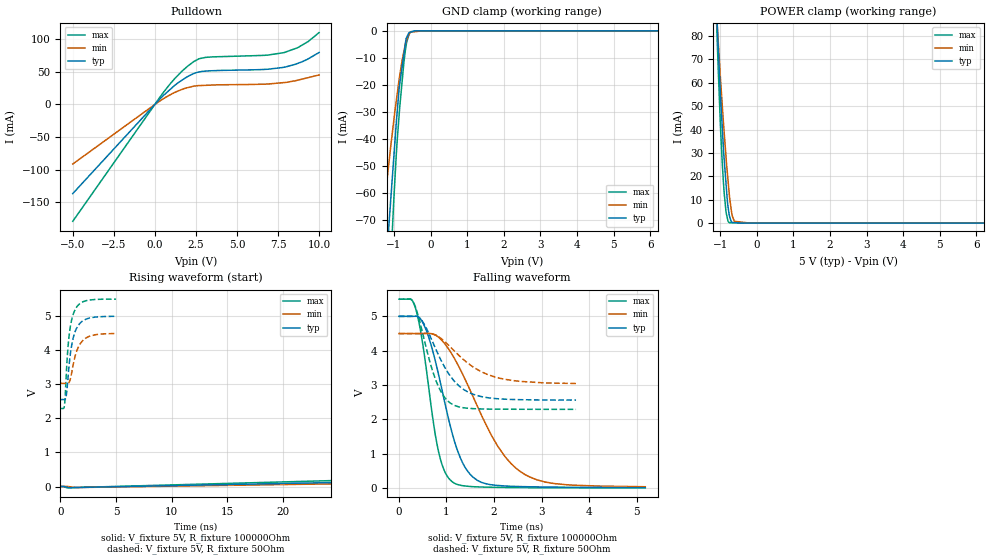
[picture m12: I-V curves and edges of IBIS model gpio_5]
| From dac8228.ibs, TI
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|   gpio_5 Model
[Model]   gpio_5
Model_type   I/O_open_drain
Polarity   Non-Inverting
Enable   Active-Low
Vinl = 0.8
Vinh = 3.8
Vmeas = 2.25
Vref = 5
Cref = 10pF
Rref = 100000
|   typ   min   max
|   (nom PVT)   (Fast PVT)   (slow PVT)
|C_comp from frequency method(F=50MHz)
|Average
C_comp   7.613e-12   6.267e-12   8.966e-12
|ON state : BUFFER OUTPUT TURNED LOW
|C_comp   7.719e-12   6.391e-12   9.083e-12
|OFF state: BUFFER IN HIGH IMPEDANCE
|C_comp   7.508e-12   6.143e-12   8.849e-12
|C_comp from L-C Tank method(L=1nH)
|Average
|C_comp   7.024e-12   5.919e-12   8.186e-12
|ON state : BUFFER OUTPUT TURNED LOW
|Resonant Frequency(Hz)   1.890e+09   2.050e+09   1.750e+09
|C_comp   7.098e-12   6.033e-12   8.279e-12
|OFF state: BUFFER IN HIGH IMPEDANCE
|Resonant Frequency(Hz)   1.910e+09   2.090e+09   1.770e+09
|C_comp   6.950e-12   5.805e-12   8.093e-12
| Where nom  PVT is Nominal Process,  5V,  33C
|   Fast PVT is Strong Process,   5.5V,  -40C
|   Slow PVT is Weak Process,   4.5V,  113C
[Voltage Range]   5   4.5   5.5
|Ambient Temperature   25   105   -40
|Junction Temperature
[Temperature Range]   33   113   -40
[Pullup Reference]   5   4.5   5.5
[Pulldown Reference]   0   0   0
[Power Clamp Reference]   5   4.5   5.5
[GND Clamp Reference]   0   0   0
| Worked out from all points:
|   slope of the pulldown table from 0 to 0.75 V, typ, clamps not added: 39.7 ohm
|   GND clamp passes 1 mA (typ) near -0.60 V on its own axis
|   POWER clamp passes 1 mA (typ) near -0.70 V on its own axis
|   falling waveform, V_fixture 5V, R_fixture 100000Ohm: 20-80 % time 545ps typ, 991ps min, 350ps max; typ from 5 V to 0.008 V
|   rising waveform, V_fixture 5V, R_fixture 100000Ohm: 20-80 % time 1.09us typ, 1.29us min, 888ns max; typ from 0.002 V to 4.98 V
|   falling waveform, V_fixture 5V, R_fixture 50Ohm: 20-80 % time 583ps typ, 809ps min, 402ps max; typ from 5 V to 2.56 V
|   rising waveform, V_fixture 5V, R_fixture 50Ohm: 20-80 % time 636ps typ, 800ps min, 515ps max; typ from 2.55 V to 5 V
[Pulldown]
|   Voltage   I(typ)   I(min)   I(max)
-5V       -136.5mA   -91.21mA   -178.9mA
528mV     13.89mA    8.876mA    18.73mA
1.221V    29.43mA    18.44mA    39.85mA
2.007V    42.76mA    25.78mA    58.81mA
2.684V    49.65mA    28.82mA    69.89mA
3.08V     51.01mA    29.23mA    71.98mA
6.6V      53.49mA    31mA       75.06mA
7.854V    56.91mA    33.43mA    79.28mA
8.684V    62.67mA    37.04mA    86.67mA
9.345V    69.89mA    41.09mA    96.42mA
10V       79.54mA    45.11mA    110mA
[GND Clamp]
|   Voltage   I(typ)   I(min)   I(max)
-5V       -981.7mA   -687.3mA   -1.357A
-1.368V   -120.3mA   -78.69mA   -173.2mA
-1.228V   -91.1mA    -60.29mA   -129.3mA
-1.14V    -72.57mA   -49.33mA   -102.3mA
-1.089V   -62.95mA   -43.03mA   -86.87mA
-1.001V   -46.36mA   -32.99mA   -61.99mA
-929.5mV  -33.02mA   -25.32mA   -44.54mA
-855mV    -20.97mA   -17.76mA   -30.72mA
-693mV    -5.221mA   -5.274mA   -7.735mA
-670mV    -2.985mA   -4.048mA   -5.704mA
-544.5mV  -503.3uA   -473.7uA   -353.4uA
10V       0A         0A         0A
[POWER Clamp]
|   Voltage   I(typ)   I(min)   I(max)
-5V       1.399A     1.179A     1.687A
-1.111V   95.69mA    93.54mA    92.87mA
-1.056V   76.86mA    79.04mA    67.78mA
-984.5mV  52.94mA    60.5mA     39.43mA
-907.5mV  31.53mA    42.75mA    16.99mA
-836mV    16.41mA    27.83mA    4.45mA
-795mV    8.276mA    20.19mA    1.601mA
-742.5mV  2.885mA    11.14mA    115.5uA
-679.5mV  421.1uA    3.912mA    105.7uA
-612mV    201.1uA    759.8uA    95.21uA
-202.5mV  26.43nA    5.18nA     31.5uA
10V       0A         0A         0A
[Ramp]
R_load = 100000
|   typ   min   max
dV/dt_r   2.9977/1.09783e-06   2.69544/1.31745e-06   3.29874/8.92645e-07
dV/dt_f   2.99891/5.49879e-10   2.69849/1.00519e-09   3.2991/3.57406e-10
[Falling Waveform]
V_fixture = 5V
V_fixture_min = 4.5V
V_fixture_max = 5.5V
R_fixture = 100000Ohm
|   Time   V(typ)   V(min)   V(max)
0s        5V         4.5V       5.5V
350ps     5.003V     4.5V       5.232V
570ps     4.61V      4.502V     3.525V
820ps     3.385V     4.406V     1.141V
1.12ns    1.592V     3.883V     179.2mV
1.57ns    299.8mV    2.624V     35.44mV
2.08ns    70.83mV    1.212V     16.27mV
2.55ns    39.48mV    479.9mV    9.502mV
3.28ns    23.31mV    124.6mV    4.571mV
5.18ns    8.48mV     34.14mV    1.684mV
[Rising Waveform]
V_fixture = 5V
V_fixture_min = 4.5V
V_fixture_max = 5.5V
R_fixture = 100000Ohm
|   Time   V(typ)   V(min)   V(max)
0s        1.778mV    2.466mV    1.463mV
150.8ns   881mV      648mV      1.22V
263.1ns   1.467V     1.101V     1.969V
507.8ns   2.46V      1.914V     3.135V
688.7ns   2.988V     2.379V     3.71V
885.5ns   3.425V     2.779V     4.158V
1.304us   4.036V     3.376V     4.737V
1.857us   4.468V     3.834V     5.113V
2.706us   4.769V     4.183V     5.351V
5.373us   4.98V      4.462V     5.491V
[Falling Waveform]
V_fixture = 5V
V_fixture_min = 4.5V
V_fixture_max = 5.5V
R_fixture = 50Ohm
|   Time   V(typ)   V(min)   V(max)
0s        5V         4.5V       5.5V
247ps     5V         4.5V       5.502V
310ps     5.001V     4.5V       5.397V
469ps     4.906V     4.5V       4.679V
759ps     4.097V     4.464V     3.2V
914ps     3.642V     4.323V     2.734V
1.073ns   3.273V     4.119V     2.479V
1.451ns   2.796V     3.634V     2.321V
2ns       2.608V     3.241V     2.296V
3.724ns   2.559V     3.043V     2.29V
[Rising Waveform]
V_fixture = 5V
V_fixture_min = 4.5V
V_fixture_max = 5.5V
R_fixture = 50Ohm
|   Time   V(typ)   V(min)   V(max)
0s        2.554V     3.029V     2.289V
356ps     2.551V     3.029V     2.364V
425ps     2.559V     3.028V     2.642V
541ps     2.704V     3.026V     3.402V
766ps     3.518V     3.051V     4.389V
1.004ns   4.135V     3.328V     4.886V
1.318ns   4.544V     3.822V     5.19V
1.726ns   4.78V      4.162V     5.362V
2.312ns   4.913V     4.362V     5.454V
4.999ns   4.996V     4.492V     5.499V
